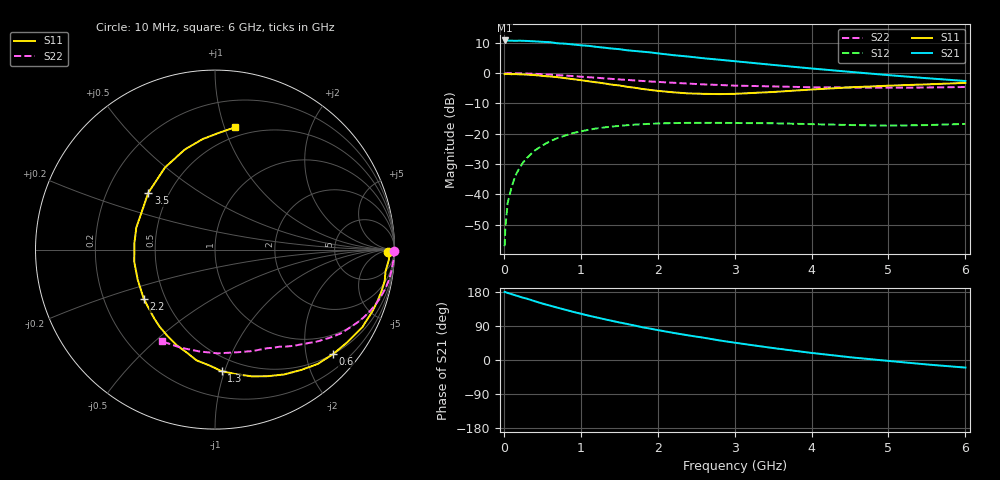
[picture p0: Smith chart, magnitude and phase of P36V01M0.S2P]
! SIEMENS Small Signal Semiconductors
! BFP181
! Si NPN RF Bipolar Junction Transistor in SOT143
! VCE = 6 V  IC = 1 mA
! Common Emitter S-Parameters:  March  1996
# GHz  S  MA  R  50
!  f  S11  S21  S12  S22
! GHz  MAG  ANG  MAG  ANG  MAG  ANG  MAG  ANG
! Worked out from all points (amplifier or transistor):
!   36 points, 10 MHz to 6 GHz, reference 50 ohm
!   highest |S21| = 10.8 dB at 10 MHz (marker M1)
!   |S21| within 3 dB of that: start of sweep to 1.537 GHz
!   unconditionally stable (mu >= 1): 3.204 GHz to end of sweep
!   at 250 MHz: K = 0.09, MSG = 20.1 dB, |S12| = -29.5 dB
!   at 1.4 GHz: K = 0.48, MSG = 12.9 dB, |S12| = -17.6 dB
!   at 6 GHz: K = 1.26, MAG = 4.0 dB, |S12| = -16.8 dB
!   lowest NFmin = 1.30 dB at 450 MHz
!   S11 on the Smith chart (normalised r, x): 10 MHz: 49, -16; 600 MHz: 0.50, -2.56; 1.3 GHz: 0.39, -0.98; 2.2 GHz: 0.38, -0.27; 3.5 GHz: 0.38, +0.32; 6 GHz: 0.42, +1.08
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0.01  0.9637 -0.7  3.454 179.6  0.0014 83.3  0.9982 -0.3
0.02  0.9721 -1.7  3.447 179.2  0.0029 90.5  0.9914 -0.6
0.05  0.9702 -3.4  3.44 176.9  0.0072 91.9  0.9961 -1.6
0.1  0.958 -7.3  3.422 173.8  0.0132 83.5  0.9963 -3.3
0.15  0.9614 -10.5  3.408 170.7  0.0205 82.7  0.9927 -5.0
0.3  0.9429 -21.1  3.389 161.9  0.0399 76.0  0.9836 -9.9
0.4  0.9274 -27.9  3.338 155.2  0.0526 71.5  0.9736 -13.0
0.6  0.8787 -41.4  3.235 143.5  0.0752 62.8  0.9446 -19.1
0.7  0.8569 -48.0  3.099 137.9  0.0851 58.5  0.9276 -21.9
0.8  0.8248 -54.4  3.053 132.5  0.0936 54.6  0.911 -24.4
1.1  0.7343 -74.0  2.815 117.1  0.1162 43.9  0.8556 -31.7
1.3  0.6787 -86.8  2.629 108.0  0.1268 37.6  0.8204 -35.9
1.5  0.626 -99.4  2.483 99.2  0.1345 32.5  0.7858 -39.5
1.8  0.5483 -119.1  2.257 86.5  0.1438 25.7  0.7422 -44.3
2.2  0.4829 -145.1  1.978 71.7  0.1499 17.8  0.6935 -50.6
2.4  0.4624 -158.6  1.873 64.9  0.151 14.3  0.6718 -53.5
2.8  0.4506 175.8  1.664 51.8  0.1511 9.3  0.6373 -59.1
3.5  0.4884 139.6  1.365 31.5  0.149 2.4  0.6031 -69.5
4  0.5358 121.3  1.192 18.7  0.144 -0.3  0.5845 -78.4
4.5  0.5825 106.8  1.049 7.3  0.1393 -2.0  0.5782 -88.4
5.5  0.6522 87.8  0.824 -11.8  0.139 0.5  0.5789 -109.2
6  0.6892 80.9  0.741 -20.0  0.1451 1.3  0.5898 -120.0
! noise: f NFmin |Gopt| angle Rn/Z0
0.45  1.3  0.7  18  0.5
0.9  1.4  0.6  39  0.52
1.8  1.85  0.4  81  0.47
